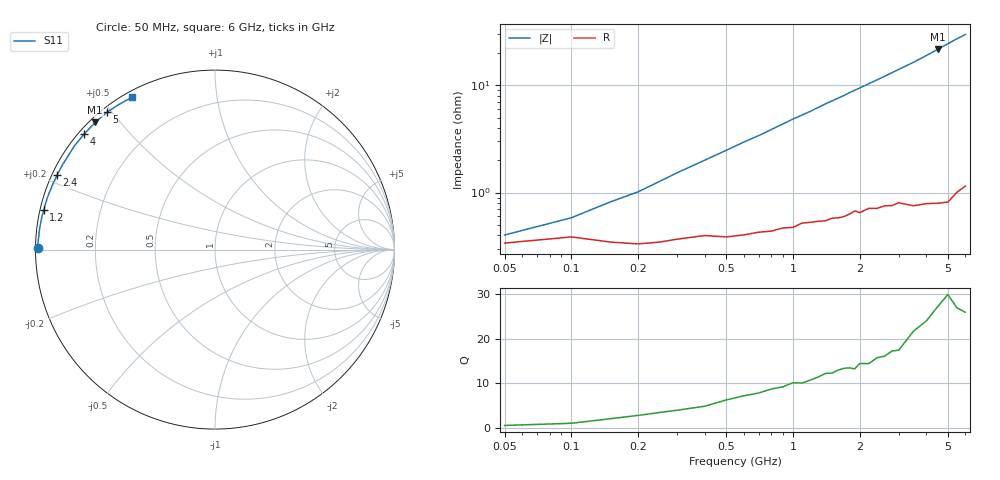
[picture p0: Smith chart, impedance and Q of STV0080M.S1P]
! SIEMENS Discrete & RF Semiconductors
! BA892
! Si PIN Diode in SCD-80
! IF = 80 mA
! S-Parameters:  September  1997
# GHz  S  MA  R  50
!  f  S11
! GHz  MAG  ANG
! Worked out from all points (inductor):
!   34 points, 50 MHz to 6 GHz, reference 50 ohm
!   read as one part to ground: L = 782 pH near 250 MHz
!   highest Q = 27.1 at 4.5 GHz (marker M1), where L = 763 pH
!   S11 on the Smith chart (normalised r, x): 50 MHz: 0.01, +0.00; 1.2 GHz: 0.01, +0.11; 2.4 GHz: 0.01, +0.22; 4 GHz: 0.02, +0.38; 5 GHz: 0.02, +0.49; 6 GHz: 0.02, +0.59
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0.05  0.9866 179.5
0.1  0.9847 179.0
0.15  0.9862 178.3
0.2  0.9868 177.8
0.3  0.9854 176.6
0.4  0.9842 175.5
0.5  0.9847 174.4
0.6  0.984 173.3
0.7  0.9831 172.3
0.8  0.9827 171.2
1  0.9814 169.0
1.1  0.9796 168.0
1.2  0.9793 167.0
1.4  0.9788 164.8
1.6  0.9775 162.8
1.7  0.9769 161.8
1.8  0.9758 160.7
1.9  0.9742 159.7
2  0.9752 158.7
2.4  0.9732 154.7
2.8  0.972 150.7
3  0.9706 148.7
3.5  0.9731 143.8
4  0.9728 138.6
4.5  0.9735 133.3
5  0.974 128.1
5.5  0.9693 123.1
6  0.9667 118.6
